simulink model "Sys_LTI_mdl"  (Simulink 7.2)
settings: Solver=ode45  StartTime=0.0  StopTime=10.0  RelTol=1e-3
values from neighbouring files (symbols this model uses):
  g = 9.81    [Esercitazione04.m]
  RispostaForzata = 1    [Esercitazione04.m]
libraries: cstblocks x1

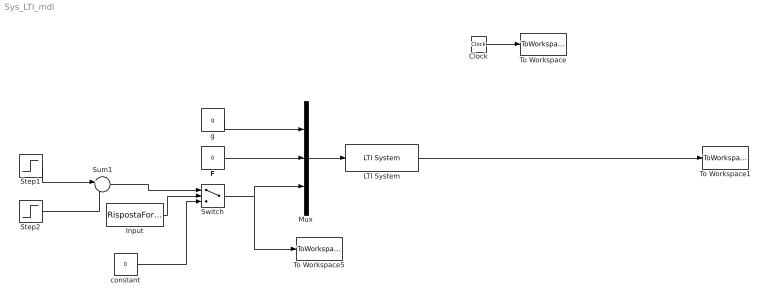
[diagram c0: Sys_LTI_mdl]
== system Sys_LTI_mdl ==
  Clock : Clock
  F : Constant  Value=0  OutDataType=sfix(16)  OutScaling=2^0
  Input : Constant  Value=RispostaForzata  OutDataType=sfix(16)  OutScaling=2^0
  LTI System : cstblocks/LTI System  SystemSampleTime=-1  sys=sys  IC=X0
  Mux : Mux  Inputs=3
  Step1 : Step  Time=5  SampleTime=0
  Step2 : Step  Time=5+0.2  SampleTime=0
  Sum1 : Sum  Inputs=+-  OutDataType=sfix(16)  OutScaling=2^0
  Switch : Switch  Threshold=0.5  OutDataType=sfix(16)  OutScaling=2^0
  To Workspace : ToWorkspace  VariableName=time  SampleTime=-1  SaveFormat=Array
  To Workspace1 : ToWorkspace  VariableName=y  SampleTime=-1  SaveFormat=Array
  To Workspace5 : ToWorkspace  VariableName=dXs  SampleTime=-1  SaveFormat=Array
  constant : Constant  Value=0  OutDataType=sfix(16)  OutScaling=2^0
  g : Constant  Value=g  OutDataType=sfix(16)  OutScaling=2^0
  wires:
  Clock/1 -> To Workspace/1
  LTI System/1 -> To Workspace1/1
  Mux/1 -> LTI System/1
  g/1 -> Mux/1
  F/1 -> Mux/2
  Switch/1 -> Mux/3, To Workspace5/1
  Step1/1 -> Sum1/1
  Step2/1 -> Sum1/2
  Sum1/1 -> Switch/1
  Input/1 -> Switch/2
  constant/1 -> Switch/3
